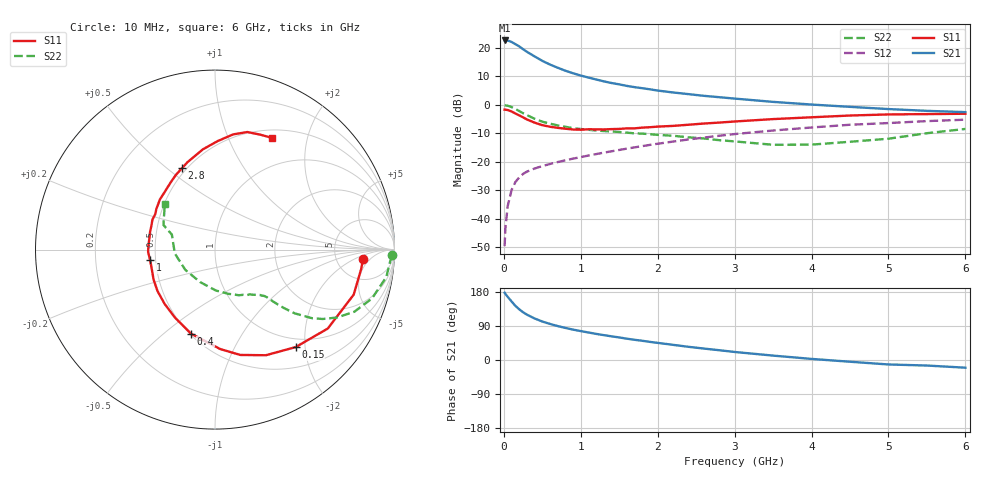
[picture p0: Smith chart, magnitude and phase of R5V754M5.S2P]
! SIEMENS Small Signal Semiconductors
! BFR183
! Si NPN RF Bipolar Junction Transistor in SOT23
! VCE = 0.75 V  IC = 4.5 mA
! Common Emitter S-Parameters:  May  1996
# GHz  S  MA  R  50
!  f  S11  S21  S12  S22
! GHz  MAG  ANG  MAG  ANG  MAG  ANG  MAG  ANG
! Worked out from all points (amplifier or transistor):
!   36 points, 10 MHz to 6 GHz, reference 50 ohm
!   highest |S21| = 22.6 dB at 10 MHz (marker M1)
!   |S21| within 3 dB of that: start of sweep to 246.2 MHz
!   unconditionally stable (mu >= 1): 984.8 MHz to 3.019 GHz
!   at 250 MHz: K = 0.40, MSG = 21.9 dB, |S12| = -24.3 dB
!   at 1.4 GHz: K = 1.08, MAG = 10.2 dB, |S12| = -16.3 dB
!   at 6 GHz: K = 0.95, MSG = 1.3 dB, |S12| = -5.2 dB
!   S11 on the Smith chart (normalised r, x): 10 MHz: 9.40, -3.15; 150 MHz: 0.84, -1.82; 400 MHz: 0.51, -0.62; 1 GHz: 0.47, -0.06; 2.8 GHz: 0.47, +0.56; 6 GHz: 0.60, +1.46
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0.01  0.8256 -3.7  13.53 177.5  0.0033 91.6  0.9868 -1.9
0.02  0.8222 -7.3  13.41 174.6  0.0068 87.8  0.9789 -3.6
0.05  0.8125 -18.0  13.48 166.7  0.0166 80.3  0.9668 -9.1
0.1  0.7669 -35.0  12.74 154.6  0.0318 72.0  0.9159 -17.3
0.15  0.705 -50.4  11.64 142.9  0.0441 65.2  0.8504 -24.0
0.2  0.6532 -64.3  10.65 133.8  0.0533 60.2  0.778 -29.1
0.25  0.6036 -76.5  9.494 126.0  0.0613 56.2  0.7138 -32.8
0.3  0.5549 -87.0  8.55 119.7  0.0673 54.2  0.6612 -35.3
0.4  0.4869 -105.9  7.092 109.6  0.0763 50.9  0.5703 -38.6
0.5  0.4402 -120.3  5.928 101.5  0.0841 49.9  0.5071 -40.2
0.6  0.413 -132.7  5.105 95.2  0.0916 49.4  0.4673 -41.1
0.7  0.3949 -144.2  4.49 89.5  0.099 49.8  0.4365 -41.7
0.8  0.3813 -153.7  3.979 84.7  0.1063 50.0  0.4117 -42.2
1  0.366 -170.8  3.274 76.3  0.1209 51.5  0.3767 -43.3
1.1  0.373 -178.0  3.017 72.6  0.129 51.8  0.3656 -44.5
1.6  0.3866 154.4  2.153 56.2  0.1706 52.1  0.325 -50.6
2.2  0.4274 130.6  1.651 40.0  0.2267 49.8  0.2867 -62.5
2.8  0.4887 112.2  1.364 25.8  0.2871 44.8  0.2397 -80.6
3.5  0.5626 96.9  1.129 11.6  0.3545 36.6  0.199 -114.7
4.5  0.65 81.0  0.923 -4.6  0.4474 23.9  0.2249 -174.5
5.5  0.6884 68.4  0.785 -14.6  0.5187 11.9  0.318 154.5
6  0.6986 63.0  0.746 -20.3  0.5495 4.0  0.3778 137.8
